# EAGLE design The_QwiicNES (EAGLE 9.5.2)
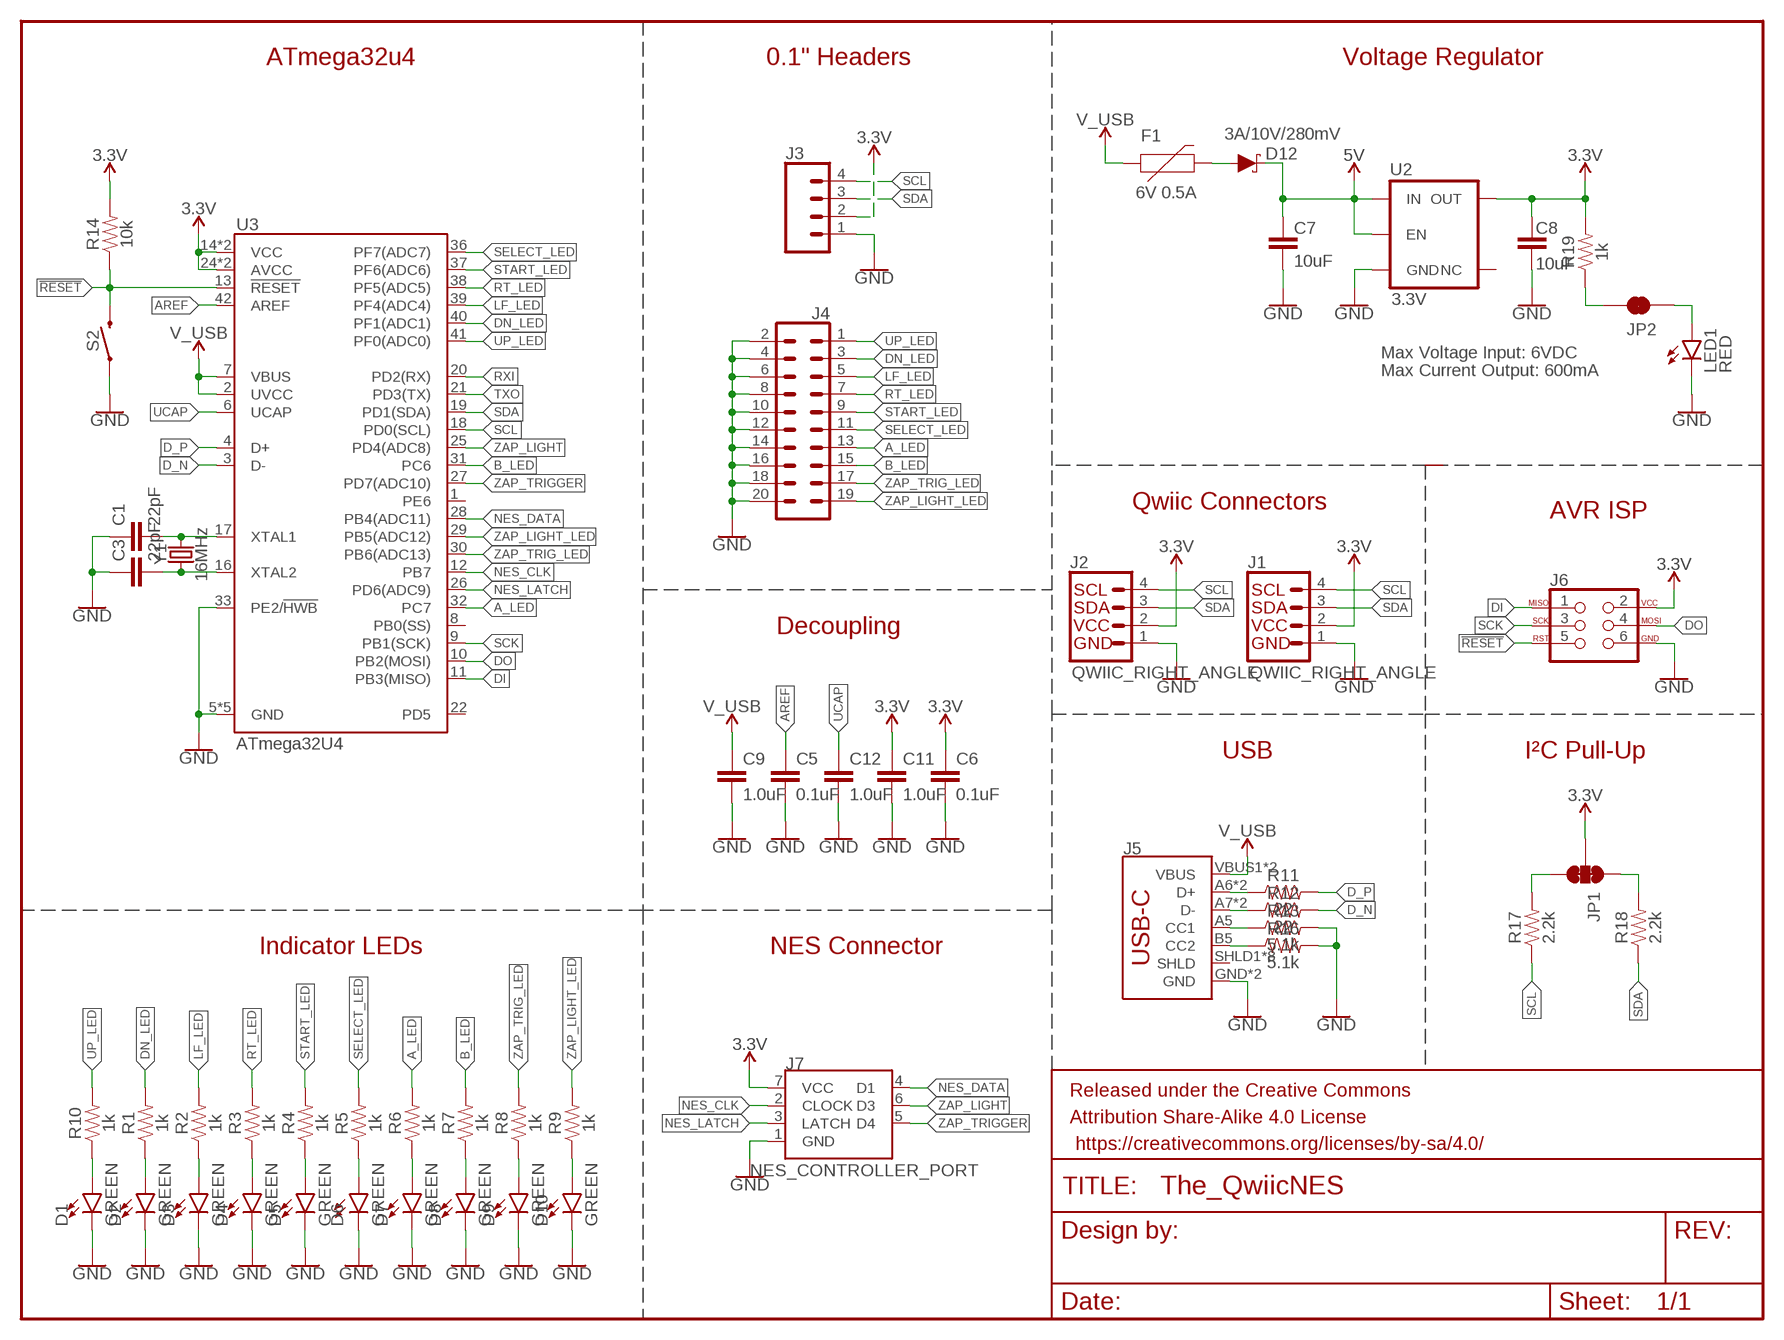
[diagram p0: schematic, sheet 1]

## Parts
C1  22pF  22PF-0603-50V-5%  [0603]
C3  22pF  22PF-0603-50V-5%  [0603]
C5  0.1uF  0.1UF-0603-25V-(+80/-20%)  [0603]
C6  0.1uF  0.1UF-0603-25V-(+80/-20%)  [0603]
C7  10uF  10UF-0603-6.3V-20%  [0603]
C8  10uF  10UF-0603-6.3V-20%  [0603]
C9  1.0uF  1.0UF-0603-16V-10%  [0603]
C11  1.0uF  1.0UF-0603-16V-10%  [0603]
C12  1.0uF  1.0UF-0603-16V-10%  [0603]
D1  GREEN  LED-GREEN0603  [LED-0603]
D2  GREEN  LED-GREEN0603  [LED-0603]
D3  GREEN  LED-GREEN0603  [LED-0603]
D4  GREEN  LED-GREEN0603  [LED-0603]
D5  GREEN  LED-GREEN0603  [LED-0603]
D6  GREEN  LED-GREEN0603  [LED-0603]
D7  GREEN  LED-GREEN0603  [LED-0603]
D8  GREEN  LED-GREEN0603  [LED-0603]
D9  GREEN  LED-GREEN0603  [LED-0603]
D10  GREEN  LED-GREEN0603  [LED-0603]
D12  3A/10V/280mV  DIODE-SCHOTTKY-BAT60A  [SOD-323]
F1  6V 0.5A  PPTC_6V500MA  [0805]
FRAME1  FRAME-LETTER  [CREATIVE_COMMONS]
J1  QWIIC_RIGHT_ANGLE  QWIIC_CONNECTORJS-1MM  [JST04_1MM_RA]
J2  QWIIC_RIGHT_ANGLE  QWIIC_CONNECTORJS-1MM  [JST04_1MM_RA]
J3  CONN_041X04_NO_SILK  [1X04_NO_SILK]
J4  CONN_10X2NOSILK  [2X10_NOSILK]
J5  USB_C5  [USB-C-16P-5]
J6  AVR_SPI_PROG_3X2TESTPOINTS  [2X3_TEST_POINTS]
J7  NES_CONTROLLER_PORT  [NES_CONTROLLER_PORT_7PIN_90]
JP1  JUMPER-SMT_3_2-NC_TRACE_SILK  [SMT-JUMPER_3_2-NC_TRACE_SILK]
JP2  JUMPER-SMT_2_NC_TRACE_SILK  [SMT-JUMPER_2_NC_TRACE_SILK]
LED1  RED  LED-RED0603  [LED-0603]
R1  1k  1KOHM-0603-1/10W-1%  [0603]
R2  1k  1KOHM-0603-1/10W-1%  [0603]
R3  1k  1KOHM-0603-1/10W-1%  [0603]
R4  1k  1KOHM-0603-1/10W-1%  [0603]
R5  1k  1KOHM-0603-1/10W-1%  [0603]
R6  1k  1KOHM-0603-1/10W-1%  [0603]
R7  1k  1KOHM-0603-1/10W-1%  [0603]
R8  1k  1KOHM-0603-1/10W-1%  [0603]
R9  1k  1KOHM-0603-1/10W-1%  [0603]
R10  1k  1KOHM-0603-1/10W-1%  [0603]
R11  22  22OHM-0603-1/10W-1%  [0603]
R12  22  22OHM-0603-1/10W-1%  [0603]
R13  5.1k  5.1KOHM5.1KOHM-0603-1/10W-1%  [0603]
R14  10k  10KOHM-0603-1/10W-1%  [0603]
R16  5.1k  5.1KOHM5.1KOHM-0603-1/10W-1%  [0603]
R17  2.2k  2.2KOHM-0603-1/10W-1%  [0603]
R18  2.2k  2.2KOHM-0603-1/10W-1%  [0603]
R19  1k  1KOHM-0603-1/10W-1%  [0603]
S2  MOMENTARY-SWITCH-SPST-SMD-5.2MM-TALL  [TACTILE_SWITCH_SMD_5.2MM]
U2  3.3V  V_REG_AP2112K-3.3V  [SOT23-5]
U3  ATmega32U4  ATMEGA32U41:1  [QFN-44-NOPAD_1:1]
Y1  16MHz  CRYSTAL-16MHZSMD-2X1.6  [CRYSTAL-SMD-2.0X1.6MM]

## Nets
3.3V: C6.1 C8.2 C11.1 J1.2 J2.2 J3.2 J6.2 J7.7(VCC) JP1.2 R14.2 R19.2 U2.5(OUT) U3.14(VCC) U3.24(AVCC) U3.34(VCC) U3.44(AVCC)
5V [vcc]: C7.2 D12.C U2.1(IN) U2.3(EN)
!RESET: J6.5 R14.1 S2.3 U3.13(!RESET)
A_LED: J4.13 R6.2 U3.32(PC7)
AREF: C5.1 U3.42(AREF)
B_LED: J4.15 R7.2 U3.31(PC6)
D-_HV: J5.A7(D-) J5.B7(D-) R12.1
D_N: R12.2 U3.3(D-)
D_P: R11.2 U3.4(D+)
DI: J6.1 U3.11(PB3(MISO))
DN_LED: J4.3 R1.2 U3.40(PF1(ADC1))
DO: J6.4 U3.10(PB2(MOSI))
DP_HV: J5.A6(D+) J5.B6(D+) R11.1
GND: C1.1 C3.1 C5.2 C6.2 C7.1 C8.1 C9.2 C11.2 C12.2 D1.C D2.C D3.C D4.C D5.C D6.C D7.C D8.C D9.C D10.C J1.1 J2.1 J3.1 J4.2 J4.4 J4.6 J4.8 J4.10 J4.12 J4.14 J4.16 J4.18 J4.20 J5.GND J5.GND2(GND) J6.6 J7.1(GND) LED1.C R13.2 R16.2 S2.1 U2.2(GND) U3.5(GND) U3.15(GND) U3.23(GND) U3.33(PE2/!HWB) U3.35(GND) U3.43(GND)
LF_LED: J4.5 R2.2 U3.39(PF4(ADC4))
N$1: C3.2 U3.16(XTAL2) Y1.1
N$2: C1.2 U3.17(XTAL1) Y1.3
N$3: D1.A R10.1
N$4: D2.A R1.1
N$5: D3.A R2.1
N$6: D4.A R3.1
N$7: D5.A R4.1
N$8: D6.A R5.1
N$9: J5.A5(CC1) R13.1
N$10: J5.B5(CC2) R16.1
N$11: D8.A R7.1
N$12: D7.A R6.1
N$13: JP2.2 R19.1
N$14: JP2.1 LED1.A
N$21: JP1.3 R17.2
N$22: JP1.1 R18.2
N$23: D10.A R9.1
N$24: D9.A R8.1
NES_CLK: J7.2(CLOCK) U3.12(PB7)
NES_DATA: J7.4(D1) U3.28(PB4(ADC11))
NES_LATCH: J7.3(LATCH) U3.26(PD6(ADC9))
RT_LED: J4.7 R3.2 U3.38(PF5(ADC5))
RXI: U3.20(PD2(RX))
SCK: J6.3 U3.9(PB1(SCK))
SCL: J1.4 J2.4 J3.4 R17.1 U3.18(PD0(SCL))
SDA: J1.3 J2.3 J3.3 R18.1 U3.19(PD1(SDA))
SELECT_LED: J4.11 R5.2 U3.36(PF7(ADC7))
START_LED: J4.9 R4.2 U3.37(PF6(ADC6))
TXO: U3.21(PD3(TX))
UCAP: C12.1 U3.6(UCAP)
UP_LED: J4.1 R10.2 U3.41(PF0(ADC0))
USB_RAW: D12.A F1.2
V_USB: C9.1 F1.1 J5.VBUS1(VBUS) J5.VBUS2(VBUS) U3.2(UVCC) U3.7(VBUS)
ZAP_LIGHT: J7.6(D3) U3.25(PD4(ADC8))
ZAP_LIGHT_LED: J4.19 R9.2 U3.29(PB5(ADC12))
ZAP_TRIG_LED: J4.17 R8.2 U3.30(PB6(ADC13))
ZAP_TRIGGER: J7.5(D4) U3.27(PD7(ADC10))
Unconnected: J5.SHLD1(SHLD) J5.SHLD2(SHLD) J5.SHLD3(SHLD) J5.SHLD4(SHLD) J5.SHLD5(SHLD) J5.SHLD6(SHLD) J5.SHLD7(SHLD) J5.SHLD8(SHLD) U2.4(NC) U3.1(PE6) U3.8(PB0(SS)) U3.22(PD5)

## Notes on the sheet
- ATmega32u4 | 0.1" Headers | Voltage Regulator
- Max Voltage Input: 6VDC
- Max Current Output: 600mA
- Qwiic Connectors
- AVR ISP
- Decoupling
- USB | I²C Pull-Up
- Indicator LEDs | NES Connector

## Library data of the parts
C1 C3 = SparkFun-Capacitors:22PF: 22pF ceramic capacitors; PROD_ID: CAP-07876
C5 C6 = SparkFun-Capacitors:0.1UF: 0.1µF ceramic capacitors; PROD_ID: CAP-00810
C7 C8 = SparkFun-Capacitors:10UF: 10.0µF ceramic capacitors; PROD_ID: CAP-11015
C9 C11 C12 = SparkFun-Capacitors:1.0UF: 1µF ceramic capacitors; PROD_ID: CAP-00868
D1-D10 = SparkFun-LED:LED-GREEN: Green SMD LED; PROD_ID: DIO-00821
D12 = SparkFun-DiscreteSemi:DIODE-SCHOTTKY: Schottky diode; PROD_ID: DIO-14072
F1 = SparkFun-Fuses:PPTC: Resettable Fuse PPTC; PROD_ID: RES-13945
FRAME1 = SparkFun-Aesthetics:FRAME-LETTER: Schematic Frame - Letter
J1 J2 = SparkFun-Connectors:QWIIC_CONNECTOR: SparkFun I2C Standard Qwiic Connector An SMD 1mm pitch JST connector makes it easy and quick (get it? Qwiic?) to connect I2C devices to each other. The Qwiic system enables fast and solderless connection between popular platforms and various sensors and actuators. We carry 200mm, 100mm, 50mm, and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; PROD_ID: CONN-13694
J3 = SparkFun-Connectors:CONN_04: Multi connection point. Often used as Generic Header-pin footprint for 0.1 inch spaced/style header connections On any of the 0.1 inch spaced packages, you can populate with these: Break Away Headers - Straight (PRT-00116) Break Away Male Headers - Right Angle (PRT-00553) Female Headers (PRT-00115)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; PROD_ID: CONN-09696
J4 = SparkFun-Connectors:CONN_10X2: Multi connection point. Often used as Generic Header-pin footprint for 0.1 inch spaced/style header connections On any of the 0.1 inch spaced packages, you can populate with these: Break Away Headers - Straight (PRT-00116) Break Away Male Headers - Right Angle (PRT-00553) Female Headers (PRT-00115)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
J5 = USBC:USB_C: USB Type C 16Pin Connector Super Speed pins not available on the 16-pin purely SMD connector so this part is best for USB 2.0 implementations. D1 and D2 are tied together enabling D+/- no matter which way the cable is plugged into the connector. The two channel configuration pins (CC1/2) are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
J6 = SparkFun-Connectors:AVR_SPI_PROG_3X2: AVR ISP 6 Pin This is the reduced ISP connector for AVR programming. Common on Arduino. This footprint will take up less PCB space and can be used with a 10-pin to 6-pin adapter such as SKU: BOB-08508 **Special note about "TEST_POINT" package. The stop mask is on the top side, so if you want your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
J7 = NES:NES_CONTROLLER_PORT
JP1 = SparkFun-Jumpers:JUMPER-SMT_3_2-NC_TRACE: Normally closed trace jumper (2 of 2 connections) This jumper has a trace between all three pads so they are normally closed (NC). Use a razor knife to open the connection(s). For best results follow the IPC guidelines for cutting traces: Cutout at least 0.063 mm (0.005 in). Remove all loose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
JP2 = SparkFun-Jumpers:JUMPER-SMT_2_NC_TRACE: Normally closed trace jumper
LED1 = SparkFun-LED:LED-RED: Red SMD LED; PROD_ID: DIO-00819
R1-R10 R19 = SparkFun-Resistors:1KOHM: 1kΩ resistor; PROD_ID: RES-07856
R11 R12 = SparkFun-Resistors:22OHM: 22Ω resistor; PROD_ID: RES-08698
R13 R16 = SparkFun-Resistors:5.1KOHM; PROD_ID: RES-12083
R14 = SparkFun-Resistors:10KOHM: 10kΩ resistor; PROD_ID: RES-00824
R17 R18 = SparkFun-Resistors:2.2KOHM: 2.2kΩ resistor; PROD_ID: RES-08272
S2 = SparkFun-Switches:MOMENTARY-SWITCH-SPST: Momentary Switch (Pushbutton) - SPST; PROD_ID: SWCH-14139
U2 = SparkFun-IC-Power:V_REG_AP2112: AP2112 - 600mA CMOS LDO Regulator w/ Enable The AP2112 is CMOS process low dropout linear regulator with enable function, the regulator delivers a guaranteed 600mA (min.) continuous load current. Features Output Voltage Accuracy: ±1.5% Output Current: 600mA (Min.) Foldback Short Current Protection: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; PROD_ID: VREG-12457
U3 = SparkFun-IC-Microcontroller:ATMEGA32U4: Atmel MCU, 32KByte Atmel 44-pin 8-bit Microcontroller with 32KBytes of ISP Flash and USB Controller Datasheet SparkFun Products LilyPad Arduino USB - ATmega32U4 Board (DEV-12049) Pro Micro - 5V/16MHz (DEV-12640) Pro Micro - 3.3V/8MHz (DEV-12587) Fio v3 - ATmega32U4 (DEV-11520) Qduino Mini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; PROD_ID: IC-10828; VALUE: 32U4
Y1 = SparkFun-Clocks:CRYSTAL-16MHZ: 16MHz Crystal; PROD_ID: XTAL-14681

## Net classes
0 default: width 0 mm, drill 0 mm

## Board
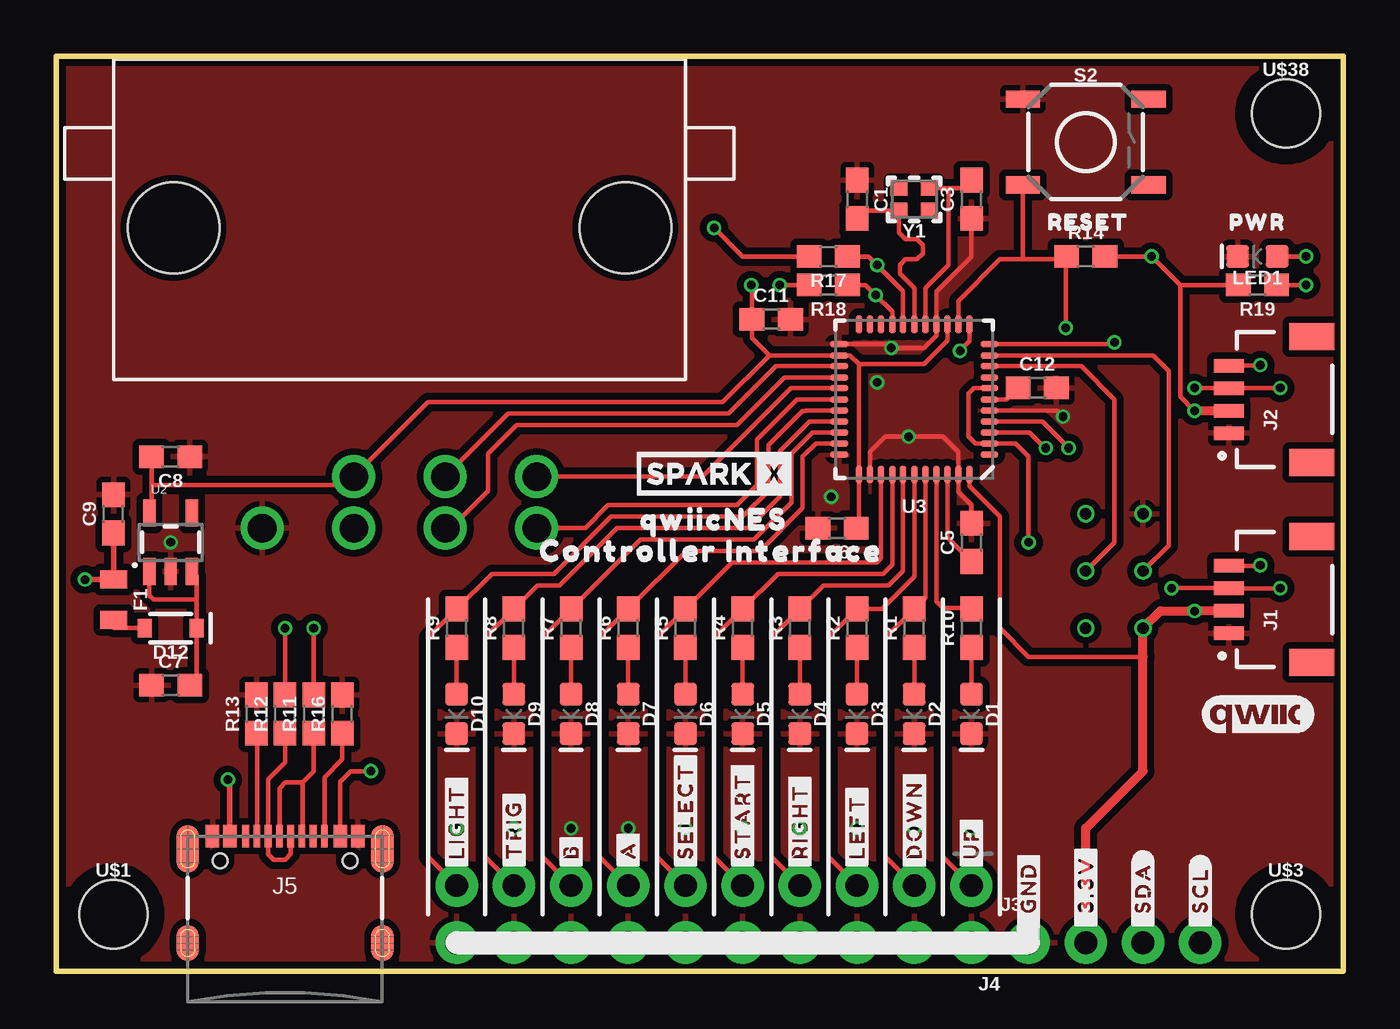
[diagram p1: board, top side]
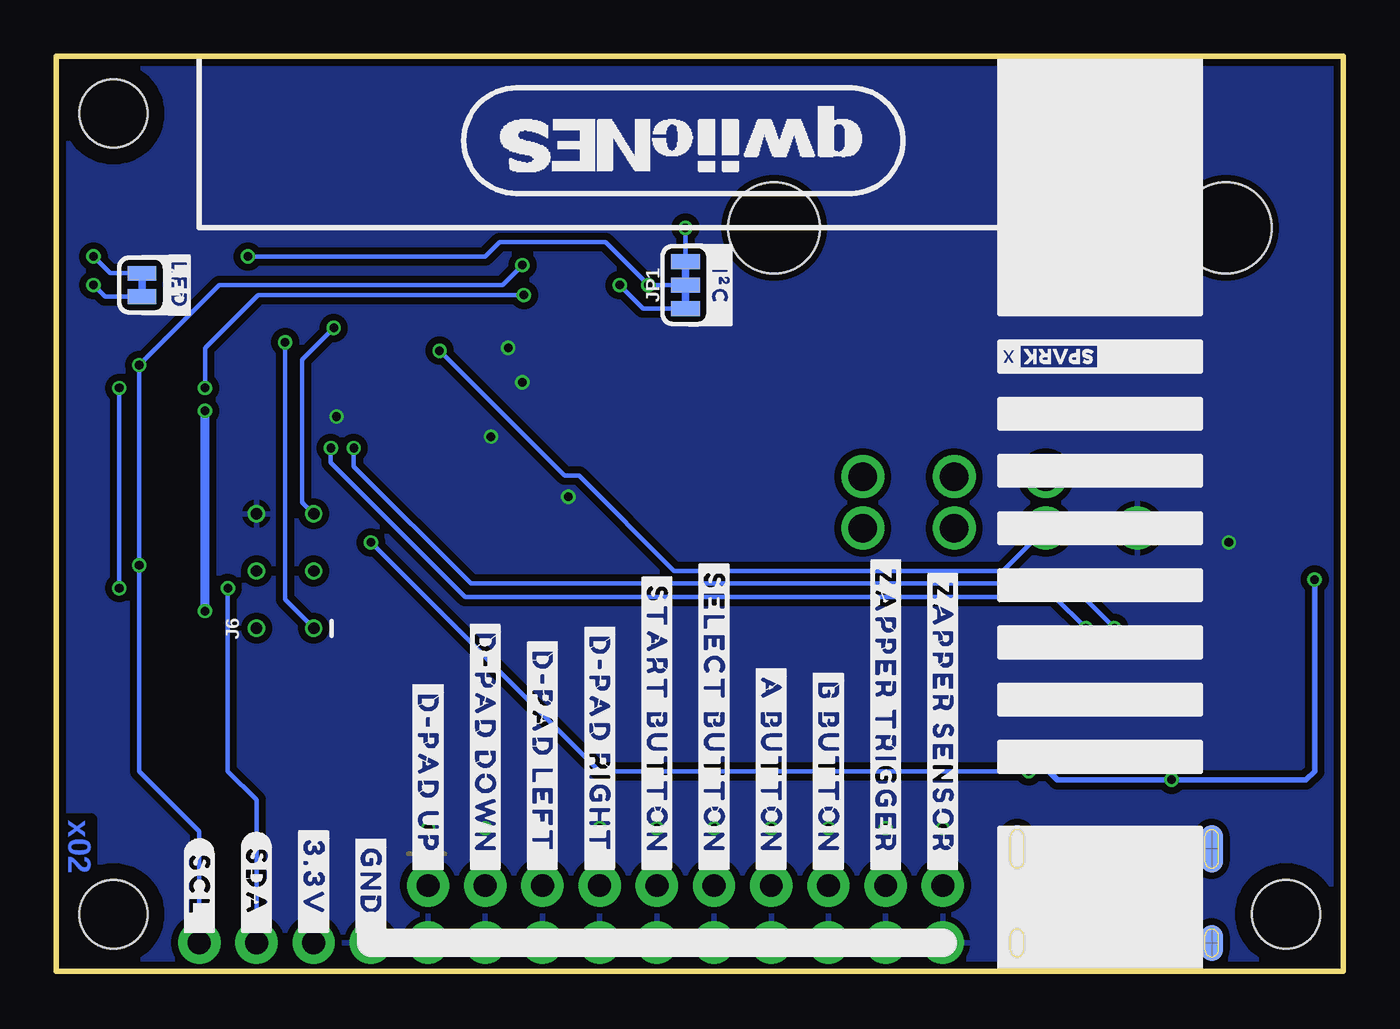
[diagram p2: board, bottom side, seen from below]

Size 57.15 x 40.64 mm. Coordinates in mm from the lower left corner, seen from the top.
Outline: 0,0 0,40.64 57.15,40.64 57.15,0 0,0
Copper layers (1*16): Top 0.035mm / dielectric 1.5mm / Bottom 0.035mm
Design rules "SparkFun-2-Layer-Minimum-JLCPCB": minimum track width 5mil, minimum drill 0.3mm, track to track 5mil, track to pad 5mil, pad to pad 5mil, via to via 5mil, smd to smd 5mil, copper to edge 7mil, drill to drill 7mil, minimum pad ring 5mil, minimum via ring 5mil, stop-mask expansion 4mil, vias tented up to drill 25mil, thermal gap 10mil

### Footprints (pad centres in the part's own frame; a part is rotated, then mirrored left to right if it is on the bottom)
0603 = smd 1.1 x 1: 1 -0.85,0; 2 0.85,0
LED-0603 = smd 1 x 1: A -0.877,0; C 0.877,0
SOD-323 = smd 0.63 x 0.83: A 1.15,0; C -1.15,0
0805 = smd 0.8 x 1.2: 1 -0.9,0; 2 0.9,0
JST04_1MM_RA = smd 0.6 x 1.35: 1 -1.5,0; 2 -0.5,0; 3 0.5,0; 4 1.5,0 | smd 1.2 x 2: NC1 2.8,-3.675; NC2 -2.8,-3.675
1X04_NO_SILK = drill 1.016 pad 1.88: 1 0,0; 2 2.54,0; 3 5.08,0; 4 7.62,0
2X10_NOSILK = drill 1.016 pad 1.88: 1 0,0; 2 0,2.54; 3 2.54,0; 4 2.54,2.54; 5 5.08,0; 6 5.08,2.54; 7 7.62,0; 8 7.62,2.54; 9 10.16,0; 10 10.16,2.54; 11 12.7,0; 12 12.7,2.54; 13 15.24,0; 14 15.24,2.54; 15 17.78,0; 16 17.78,2.54; 17 20.32,0; 18 20.32,2.54; 19 22.86,0; 20 22.86,2.54
USB-C-16P-5 = smd 0.3 x 1: A5 -1.25,-0.34; A6 -0.25,-0.34; A7 0.25,-0.34; A8 1.25,-0.34; B5 1.75,-0.34; B6 0.75,-0.34; B7 -0.75,-0.34; B8 -1.75,-0.34 | smd 0.6 x 1: GND -3.225,-0.34; GND2 3.225,-0.34; VBUS1 -2.45,-0.34; VBUS2 2.45,-0.34 | smd 1 x 2.1: SHLD1 -4.32,-0.915; SHLD2 4.32,-0.915 | smd 1 x 2.1 bottom: SHLD3 -4.32,-0.915; SHLD4 4.32,-0.915 | smd 1 x 1.6: SHLD5 -4.32,-5.095; SHLD8 4.32,-5.095 | smd 1 x 1.6 bottom: SHLD6 -4.32,-5.095; SHLD7 4.32,-5.095 | hole 0.65: -2.89,-1.445; 2.89,-1.445
2X3_TEST_POINTS = drill 0.508: 1 -2.54,-1.27; 2 -2.54,1.27; 3 0,-1.27; 4 0,1.27; 5 2.54,-1.27; 6 2.54,1.27
NES_CONTROLLER_PORT_7PIN_90 = drill 1.27: 1 -6.096,-13.335; 2 -2.032,-13.335; 3 2.032,-13.335; 4 6.096,-13.335; 5 6.096,-11.049; 6 2.032,-11.049; 7 -2.032,-11.049 | hole 4.064: -10.033,0; 10.033,0
SMT-JUMPER_3_2-NC_TRACE_SILK = smd 0.66 x 1.27: 1 -1.041,0; 2 0,0; 3 1.041,0
SMT-JUMPER_2_NC_TRACE_SILK = smd 0.66 x 1.27: 1 -0.521,0; 2 0.521,0
TACTILE_SWITCH_SMD_5.2MM = smd 1.524 x 0.762: 1 -2.794,1.905; 2 2.794,1.905; 3 -2.794,-1.905; 4 2.794,-1.905
SOT23-5 = smd 0.55 x 1.2: 1 -0.95,-1.3; 2 0,-1.3; 3 0.95,-1.3; 4 0.95,1.3; 5 -0.95,1.3
QFN-44-NOPAD_1:1 = smd 0.8 x 0.3: 1 -3.337,2.458; 2 -3.337,1.958; 3 -3.337,1.479; 4 -3.337,0.979; 5 -3.337,0.5; 6 -3.337,0; 7 -3.337,-0.5; 8 -3.337,-0.979; 9 -3.337,-1.479; 10 -3.337,-1.958; 11 -3.337,-2.458; 23 3.337,-2.458; 24 3.337,-1.958; 25 3.337,-1.479; 26 3.337,-0.979; 27 3.337,-0.5; 28 3.337,0; 29 3.337,0.5; 30 3.337,0.979; 31 3.337,1.479; 32 3.337,1.958; 33 3.337,2.458 | smd 0.3 x 0.8: 12 -2.458,-3.337; 13 -1.958,-3.337; 14 -1.479,-3.337; 15 -0.979,-3.337; 16 -0.5,-3.337; 17 0,-3.337; 18 0.5,-3.337; 19 0.979,-3.337; 20 1.479,-3.337; 21 1.958,-3.337; 22 2.458,-3.337; 34 2.458,3.337; 35 1.958,3.337; 36 1.479,3.337; 37 0.979,3.337; 38 0.5,3.337; 39 0,3.337; 40 -0.5,3.337; 41 -0.979,3.337; 42 -1.479,3.337; 43 -1.958,3.337; 44 -2.458,3.337
STAND-OFF-TIGHT = hole 3.048: 0,0
CRYSTAL-SMD-2.0X1.6MM = smd 0.75 x 0.7: 1 -0.675,-0.5; 2 0.675,-0.5; 3 0.675,0.5; 4 -0.675,0.5

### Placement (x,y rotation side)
C1  35.56,34.29 270 top
C3  40.64,34.29 90 top
C5  40.64,19.05 90 top
C6  34.67,19.68 180 top
C7  5.08,12.7 0 top
C8  5.08,22.86 180 top
C9  2.54,20.32 90 top
C11  31.75,28.96 0 top
C12  43.56,25.91 0 top
D1  40.64,11.43 270 top
D2  38.1,11.43 270 top
D3  35.56,11.43 270 top
D4  33.02,11.43 270 top
D5  30.48,11.43 270 top
D6  27.94,11.43 270 top
D7  25.4,11.43 270 top
D8  22.86,11.43 270 top
D9  20.32,11.43 270 top
D10  17.78,11.43 270 top
D12  5.08,15.24 180 top
F1  2.54,16.51 270 top
FRAME1  not placed on the board
J1  52.07,16.51 90 top
J2  52.07,25.4 90 top
J3  43.18,1.27 0 top
J4  40.64,3.81 180 top
J5  10.16,6.35 0 top
J6  46.99,17.78 90 bottom
J7  15.24,33.02 0 top
JP1  29.21,30.48 90 bottom
JP2  53.34,30.48 270 bottom
LED1  53.34,31.75 180 top
R1  38.1,15.24 90 top
R2  35.56,15.24 90 top
R3  33.02,15.24 90 top
R4  30.48,15.24 90 top
R5  27.94,15.24 90 top
R6  25.4,15.24 90 top
R7  22.86,15.24 90 top
R8  20.32,15.24 90 top
R9  17.78,15.24 90 top
R10  40.64,15.24 90 top
R11  11.43,11.43 90 top
R12  10.16,11.43 90 top
R13  8.89,11.43 90 top
R14  45.72,31.75 0 top
R16  12.7,11.43 90 top
R17  34.29,31.75 180 top
R18  34.29,30.48 180 top
R19  53.34,30.48 180 top
S2  45.72,36.83 0 top
U2  5.08,19.05 0 top
U3  38.1,25.4 180 top
U$1  [STAND-OFF-TIGHT]  2.54,2.54 0 top
U$2  [SPARKX-SMALL]  29.21,22.1 0 top
U$3  [STAND-OFF-TIGHT]  54.61,2.54 0 top
U$4  [#LIGHT#0]  17.78,4.45 90 top
U$5  [#TRIG#0]  20.32,4.45 90 top
U$6  [#B#0]  22.86,4.45 90 top
U$7  [#A#0]  25.4,4.45 90 top
U$8  [#SELECT#0]  27.94,4.45 90 top
U$9  [#START#0]  30.48,4.45 90 top
U$10  [#RIGHT#0]  33.02,4.45 90 top
U$11  [#LEFT#0]  35.56,4.45 90 top
U$12  [#DOWN#0]  38.1,4.45 90 top
U$13  [#UP#0]  40.64,4.45 90 top
U$14  [#_GND#0]  43.18,1.78 90 top
U$15  [#_SDA#0]  48.26,1.78 90 top
U$16  [#_SCL#0]  50.8,1.78 90 top
U$17  [#_3#3V#0]  45.72,1.78 90 top
U$18  [PWR0]  53.34,33.27 0 top
U$19  [RESET0]  45.85,33.27 0 top
U$20  [SPARKX-TINY]  13.08,27.3 180 bottom
U$21  [#ZAPPER_SENSOR_#0]  17.78,4.19 270 bottom
U$22  [#ZAPPER_TRIGGER_#0]  20.32,4.19 270 bottom
U$23  [#B_BUTTON_#0]  22.86,4.19 270 bottom
U$24  [#A_BUTTON_#0]  25.4,4.19 270 bottom
U$25  [#SELECT_BUTTON_#0]  27.94,4.19 270 bottom
U$26  [#START_BUTTON_#0]  30.48,4.19 270 bottom
U$27  [#D#PAD_RIGHT_#0]  33.02,4.19 270 bottom
U$28  [#D#PAD_LEFT_#0]  35.56,4.19 270 bottom
U$29  [#D#PAD_DOWN_#0]  38.1,4.19 270 bottom
U$30  [#D#PAD_UP_#0]  40.64,4.19 270 bottom
U$31  [#GND_#0]  43.18,1.4 270 bottom
U$32  [#SDA_#0]  48.26,1.4 270 bottom
U$33  [#SCL_#0]  50.8,1.4 270 bottom
U$34  [#3#3V_#0]  45.72,1.4 270 bottom
U$35  [#I�C#0]  27.69,29.08 270 bottom
U$36  [#LED#0]  51.69,30.48 270 bottom
U$37  [QWIICNESS#PNG]  29.21,36.83 180 bottom
U$38  [STAND-OFF-TIGHT]  54.61,38.1 0 top
U$39  [QWIICNES0]  29.21,20.07 0 top
U$40  [CONTROLLER_INTERFACE0]  29.08,18.67 0 top
U$41  [QWIIC_5MM]  53.34,11.43 0 top
Y1  38.1,34.29 180 top

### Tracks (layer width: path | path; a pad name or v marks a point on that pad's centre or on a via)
3.3V  (via drill 0.38)
  Top 0.203: U3.14 39.58,28.02 38.53,26.97 35.64,26.97 | 35.64,26.97 U3.34 35.64,19.81 C6.1 | 35.64,26.97 35.25,27.36 U3.24 31.68,27.36 | C8.2 4.23,21.59 | 4.23,21.59 4.23,20.45 U2.5 | 31.68,27.36 29.59,25.27 16.51,25.27 J7.7 12.83,21.59 4.23,21.59 | v50.55,24.89 49.91,25.53 49.91,30.48 | U3.44 40.56,21.55 41.91,20.19 41.91,15.24 43.18,13.97 48.26,13.97 | v30.86,30.48 30.9,30.44 C11.1 30.9,28.13 31.68,27.36 | R14.2 v48.64,31.75 49.91,30.48 | 49.91,30.48 R19.2
  Top 0.406: J1.2 v50.55,16.01 | v50.55,16.01 v50.55,16 | v50.55,24.89 v50.55,24.9 J2.2 | v50.55,16.01 49.03,16.01 J6.2 48.26,13.97 48.26,8.89 45.72,6.35 J3.2
  Bottom 0.203: JP1.2 v30.86,30.48 32.77,32.38 37.47,32.38 38.1,31.75 v48.64,31.75
  Bottom 0.406: v50.55,16 v50.55,24.89
5V
  Top 0.203: U2.3 6.23,17.55 6.23,16.51 | 6.23,16.51 D12.C 6.23,13 C7.2 | U2.1 4.13,16.7 4.32,16.51 6.23,16.51
!RESET  (via drill 0.38)
  Top 0.203: U3.13 40.06,29.77 41.91,31.62 42.93,31.62 | S2.3 42.93,31.62 | R14.1 44.74,31.62 | 44.74,31.62 42.93,31.62 | v44.83,28.57 44.83,31.54 44.74,31.62
  Bottom 0.203: J6.5 46.23,20.83 46.23,27.18 v44.83,28.57
A_LED
  Top 0.203: U3.32 33.73,23.44 33.15,22.86 33.15,20.57 31.24,18.67 27.98,18.67 R6.2 24.13,14.82 24.13,5.08 J4.13
AREF
  Top 0.203: U3.42 39.58,19.26 C5.1
B_LED
  Top 0.203: U3.31 33.57,23.92 32.64,22.99 32.64,20.83 30.99,19.18 25.95,19.18 R7.2 21.59,14.82 21.59,5.08 J4.15
D-_HV
  Top 0.203: J5.A7 10.41,5.21 10.16,4.95 9.65,4.95 9.41,5.2 J5.B7 9.41,8.52 10.16,9.27 R12.1
D_N  (via drill 0.38)
  Top 0.203: U3.3 43.22,23.92 43.9,23.24 v43.94,23.24 | v10.16,15.24 R12.2
  Bottom 0.203: v43.94,23.24 43.94,22.43 38.73,17.22 12.14,17.22 v10.16,15.24
D_P  (via drill 0.38)
  Top 0.203: U3.4 43.79,24.42 44.96,23.25 v44.96,23.24 | v11.43,15.24 R11.2
  Bottom 0.203: v44.96,23.24 44.96,22.61 44.27,21.92 44.27,21.91 39,16.64 12.83,16.64 v11.43,15.24
DI  (via drill 0.38)
  Top 0.203: v46.99,27.94 46.91,27.86 U3.11
  Bottom 0.203: v46.99,27.94 46.99,16.51 J6.1
DN_LED
  Top 0.203: J4.3 36.83,5.08 36.83,14.82 R1.2 38.6,16.59 U3.40
DO
  Top 0.203: J6.4 49.4,18.92 49.4,26.67 48.72,27.36 U3.10
DP_HV
  Top 0.203: 10.93,8.38 10.93,6.03 J5.B6 | J5.A6 9.91,8.13 10.16,8.38 10.93,8.38 | 10.93,8.38 11.43,8.88 R11.1
GND  (via drill 0.38)
  Top 0.203: U3.23 36.91,27.86 v37.08,27.69 38.52,27.69 39.08,28.24 U3.15 39.08,30.19 40.64,31.75 C3.1 | U3.35 36.14,23.06 36.83,23.75 v37.85,23.75 39.37,23.75 40.06,23.06 U3.43 40.06,21.28 40.64,20.7 C5.2 | v44.7,24.64 44.44,24.9 U3.5
  other vias: 5.08,19.05 34.42,21.08 36.45,26.16 40.64,6.35 38.1,6.35 35.56,6.35 33.02,6.35 30.48,6.35 27.94,6.35 25.4,6.35 22.86,6.35 20.32,6.35 17.78,6.35
  pour Top (isolate 0.305): 0,0 57.15,0 57.15,40.64 0,40.64
  pour Bottom (isolate 0.305): 0,0 57.15,0 57.15,40.64 0,40.64
LF_LED
  Top 0.203: U3.39 38.1,17.53 36.66,16.09 R2.2 34.29,14.82 34.29,5.08 J4.5
N$1
  Top 0.203: U3.16 38.6,30.34 39.62,31.37 39.62,34.79 | Y1.1 39.62,34.79 | 39.62,34.79 40.29,34.79 C3.2
N$2
  Top 0.203: C1.2 35.91,33.79 Y1.3 37.42,32.81 37.72,32.51 38.23,32.51 38.48,32.26 38.48,31.88 38.23,31.62 37.72,31.62 37.47,31.37 37.47,30.99 38.1,30.35 U3.17
N$3
  Top 0.203: R10.1 D1.A
N$4
  Top 0.203: R1.1 D2.A
N$5
  Top 0.203: R2.1 D3.A
N$6
  Top 0.203: R3.1 D4.A
N$7
  Top 0.203: R4.1 D5.A
N$8
  Top 0.203: R5.1 D6.A
N$9
  Top 0.203: R13.1 8.91,10.56 J5.A5
N$10
  Top 0.203: J5.B5 11.91,8.62 12.7,9.41 R16.1
N$11
  Top 0.203: D8.A R7.1
N$12
  Top 0.203: R6.1 D7.A
N$13  (via drill 0.38)
  Top 0.203: R19.1 v55.5,30.48
  Bottom 0.203: v55.5,30.48 54.98,29.96 JP2.2
N$14  (via drill 0.38)
  Top 0.203: LED1.A v55.5,31.75
  Bottom 0.203: v55.5,31.75 54.75,31 JP2.1
N$21  (via drill 0.38)
  Top 0.203: v29.21,33.02 30.48,31.75 R17.2
  Bottom 0.203: v29.21,33.02 JP1.3
N$22  (via drill 0.38)
  Top 0.203: R18.2 v32.13,30.48
  Bottom 0.203: v32.13,30.48 31.09,29.44 JP1.1
N$23
  Top 0.203: D10.A R9.1
N$24
  Top 0.203: D9.A R8.1
NES_CLK  (via drill 0.38)
  Top 0.203: U3.12 40.56,27.98 v40.13,27.56
  Bottom 0.203: v40.13,27.56 34.58,22.01 33.94,22.01 29.71,17.78 15.11,17.78 J7.2
NES_DATA
  Top 0.203: J7.4 23.5,19.68 24.51,20.7 30.23,20.7 31.11,21.59 31.11,23.62 32.89,25.4 U3.28
NES_LATCH
  Top 0.203: J7.3 17.53,19.68 19.18,21.34 19.18,22.99 20.45,24.26 30.23,24.26 32.35,26.38 U3.26
RT_LED
  Top 0.203: U3.38 37.6,17.79 36.96,17.14 34.08,17.14 R3.2 31.75,14.82 31.75,5.08 J4.7
SCK
  Top 0.203: J6.3 46.99,19.05 46.99,25.4 45.51,26.88 U3.9
SCL  (via drill 0.38)
  Top 0.203: J1.4 53.44,18.01 v53.47,18.03 | v53.47,26.92 53.44,26.9 J2.4 | U3.18 37.6,30.22 v36.45,31.37 36.07,31.75 R17.1
  Bottom 0.203: v36.45,31.37 37.34,30.48 49.91,30.48 v53.47,26.92 v53.47,18.03 53.47,8.89 50.8,6.22 J3.4
SDA  (via drill 0.38)
  Top 0.203: v54.36,17.02 54.35,17.01 J1.3 v49.53,17.02 | v54.36,25.91 54.35,25.9 J2.3 v50.55,25.91 | U3.19 37.12,29.3 v36.39,30.04 35.94,30.48 R18.1
  Bottom 0.203: v54.36,17.02 v54.36,25.91 | v36.39,30.04 48.2,30.04 50.55,27.69 v50.55,25.91 | v49.53,17.02 49.53,8.89 48.26,7.62 J3.3
SELECT_LED
  Top 0.203: U3.36 36.62,18.33 36.45,18.16 30.01,18.16 R5.2 26.67,14.82 26.67,5.08 J4.11
START_LED
  Top 0.203: U3.37 37.12,18.07 36.7,17.65 32.04,17.65 R4.2 29.21,14.82 29.21,5.08 J4.9
UCAP
  Top 0.203: U3.6 42.2,25.4 C12.1
UP_LED
  Top 0.203: U3.41 39.08,16.42 39.37,16.13 | J4.1 39.37,5.08 39.37,16.13 | R10.2 40.6,16.13 39.37,16.13
USB_RAW
  Top 0.203: F1.2 2.54,15.24 D12.A
V_USB  (via drill 0.38)
  Top 0.203: U3.7 40.76,25.9 40.51,25.65 40.51,23.75 40.82,23.44 U3.2 42.6,23.44 43.18,22.86 v43.18,19.05 | v13.97,8.89 13.08,8.89 12.61,8.42 J5.VBUS2
  Top 0.254: J5.VBUS1 7.71,8.42 v7.62,8.51 | v1.27,17.4 v1.28,17.41 F1.1 C9.1
  Bottom 0.203: v43.18,19.05 33.02,8.89 v13.97,8.89
  Bottom 0.254: v1.27,17.4 1.27,8.89 1.65,8.51 v7.62,8.51 12.7,8.51 13.08,8.89 v13.97,8.89
ZAP_LIGHT
  Top 0.203: J7.6 20.07,24.77 29.84,24.77 31.96,26.88 U3.25
ZAP_LIGHT_LED
  Top 0.203: U3.29 33.28,24.9 33.27,24.89 33.15,24.89 31.62,23.37 31.62,21.34 30.48,20.19 24.64,20.19 22.1,17.65 19.34,17.65 R9.2 16.51,14.82 16.51,5.08 J4.19
ZAP_TRIG_LED
  Top 0.203: U3.30 33.44,24.42 32.13,23.11 32.13,21.08 30.73,19.68 24.89,19.68 22.35,17.14 21.38,17.14 R8.2 19.05,14.82 19.05,5.08 J4.17
ZAP_TRIGGER
  Top 0.203: J7.5 28.7,21.97 32.63,25.9 U3.27

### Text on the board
Bottom: x02
tDocu: NPOOLE

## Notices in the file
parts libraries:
SparkFun-IC-Microcontroller: Licensing: Creative Commons ShareAlike 4.0 International - https://creativecommons.org/licenses/by-sa/4.0
SparkFun-Aesthetics: Released under the Creative Commons Attribution Share-Alike 4.0 License
SparkFun-Aesthetics: https://creativecommons.org/licenses/by-sa/4.0
